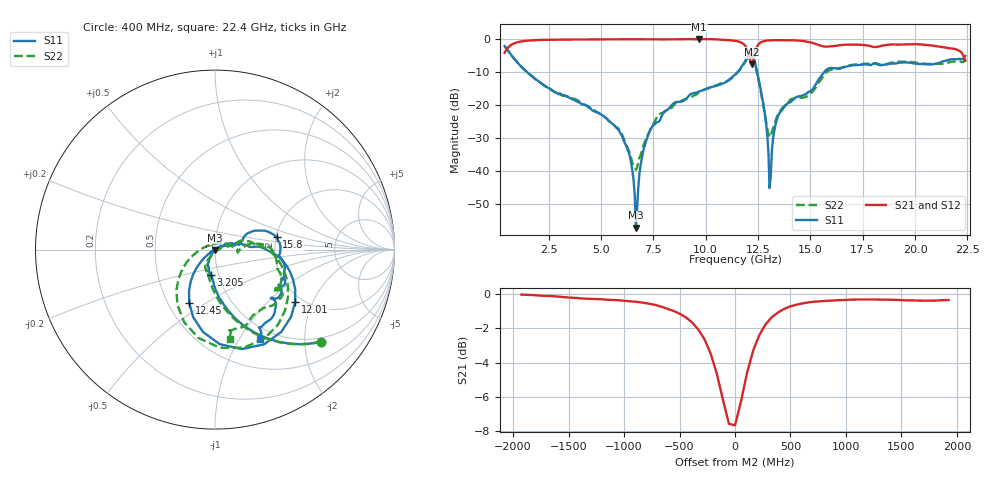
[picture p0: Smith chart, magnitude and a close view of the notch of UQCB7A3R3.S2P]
!  Part Number  UQCB7A3R3	Mounting Orientation: Vertical
!  Description: RF capacitors
!  Application: Coupling, Bypass, Tuning, DC Block
!  Filters, Matching
# GHZ S DB R 50
! Freq  |S11|  S11 Ph  |S21|  S21 Ph  |S12|  S12 Ph  |S22|  S22 Ph
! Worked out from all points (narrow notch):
!   401 points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, 400 MHz to 22.4 GHz, reference 50 ohm
!   highest |S21| = 0.00 dB at 9.695 GHz (marker M1); lowest = -7.7 dB at 12.22 GHz (marker M2)
!   notch at M2: 7.3 dB deep, 324 MHz wide at half that depth
!   lowest |S11| = -57.1 dB at 6.67 GHz (marker M3), VSWR 1.00, Z = 50 - j0.134 ohm
!   |S11| at or under -10 dB: 1.469 GHz to 11.53 GHz (10.06 GHz wide, 155 % of centre); 12.46 GHz to 15.66 GHz (3.201 GHz wide, 22.8 % of centre)
!   |S22| runs from -39.6 to -2.1 dB; largest |S21 - S12| = 0.0049
!   S11 on the Smith chart (normalised r, x): 400 MHz: 0.90, -2.39; 3.205 GHz: 0.92, -0.26; 12.01 GHz: 1.82, -1.49; 12.45 GHz: 0.64, -0.43; 15.8 GHz: 2.01, +0.31; 22.4 GHz: 0.85, -1.23
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0.4  -2.12 -41.0  -4.15 48.8  -4.18 48.8  -2.14 -41.2
1.28  -8.88 -76.8  -0.63 12.3  -0.65 12.2  -8.90 -78.1
3.205  -16.99 -99.8  -0.17 -14.4  -0.19 -14.4  -17.23 -105.2
4.085  -19.70 -110.0  -0.14 -22.6  -0.16 -22.5  -19.40 -121.1
5.9  -28.19 -126.3  -0.07 -37.7  -0.08 -37.6  -27.93 -121.0
6.395  -35.98 -125.8  -0.05 -41.8  -0.05 -41.7  -34.75 -102.6
6.67  -57.15 -75.0  -0.04 -44.1  -0.04 -44.0  -39.58 -43.6
7.11  -31.80 33.5  -0.05 -47.8  -0.05 -47.8  -31.04 9.9
7.77  -25.03 24.1  -0.08 -53.2  -0.07 -53.1  -22.75 15.5
9.695  -15.88 9.9  0.00 -69.2  -0.01 -69.1  -16.19 19.2
11.4  -10.77 -0.4  -0.50 -90.5  -0.50 -90.5  -10.97 1.1
12.005  -5.45 -33.3  -3.46 -108.1  -3.46 -108.2  -5.73 -40.9
12.225  -4.82 -75.0  -7.67 -77.5  -7.67 -77.5  -5.23 -87.0
12.445  -9.63 -115.8  -2.38 -64.3  -2.38 -64.4  -10.14 -133.7
13.105  -41.83 39.0  -0.37 -85.3  -0.36 -85.3  -29.41 83.8
13.325  -26.24 23.3  -0.31 -88.8  -0.31 -89.0  -24.88 37.7
13.545  -22.28 15.6  -0.32 -92.0  -0.32 -92.0  -21.83 19.8
15.085  -15.35 22.2  -1.13 -111.3  -1.12 -111.5  -16.04 4.7
15.8  -9.11 11.2  -2.30 -110.5  -2.28 -110.5  -9.87 -1.0
18.77  -7.52 -29.2  -1.69 -126.2  -1.66 -126.4  -7.31 -31.2
20.97  -7.49 -40.4  -2.08 -152.7  -2.07 -152.9  -7.52 -55.7
22.4  -5.08 -63.2  -6.56 -174.8  -6.58 -175.0  -5.94 -80.8
